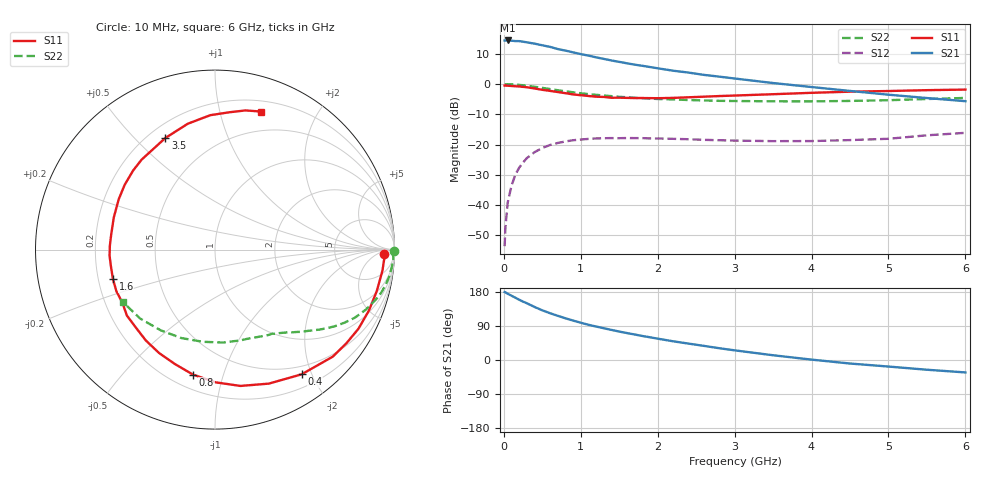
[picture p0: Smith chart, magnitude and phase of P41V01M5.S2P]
! SIEMENS Small Signal Semiconductors
! BFP182
! Si NPN RF Bipolar Junction Transistor in SOT143
! VCE = 1 V  IC = 1.5 mA
! Common Emitter S-Parameters:  March  1996
# GHz  S  MA  R  50
!  f  S11  S21  S12  S22
! GHz  MAG  ANG  MAG  ANG  MAG  ANG  MAG  ANG
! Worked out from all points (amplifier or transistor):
!   36 points, 10 MHz to 6 GHz, reference 50 ohm
!   highest |S21| = 14.4 dB at 50 MHz (marker M1)
!   |S21| within 3 dB of that: start of sweep to 732.6 MHz
!   unconditionally stable (mu >= 1): 2.318 GHz to end of sweep
!   at 250 MHz: K = 0.12, MSG = 20.0 dB, |S12| = -25.9 dB
!   at 1.4 GHz: K = 0.63, MSG = 12.8 dB, |S12| = -17.8 dB
!   at 6 GHz: K = 1.13, MAG = 3.1 dB, |S12| = -16.1 dB
!   S11 on the Smith chart (normalised r, x): 10 MHz: 29, -13; 400 MHz: 0.38, -1.85; 800 MHz: 0.29, -0.80; 1.6 GHz: 0.26, -0.13; 3.5 GHz: 0.27, +0.62; 6 GHz: 0.30, +1.35
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0.01  0.9437 -1.5  5.24 179.3  0.0021 89.0  0.9966 -0.6
0.02  0.9444 -3.0  5.253 178.6  0.0042 86.7  0.9914 -1.2
0.05  0.9403 -7.2  5.259 174.8  0.011 87.3  0.9954 -3.0
0.1  0.9305 -14.4  5.21 169.6  0.0211 80.9  0.9892 -5.9
0.2  0.9128 -28.9  5.129 159.0  0.0417 73.1  0.9709 -11.7
0.25  0.8989 -35.6  5.014 154.0  0.0507 68.4  0.9562 -14.6
0.4  0.8461 -55.2  4.653 139.9  0.0751 57.7  0.9037 -21.8
0.5  0.8047 -68.1  4.376 131.1  0.0881 50.7  0.8663 -26.0
0.6  0.7728 -79.4  4.123 123.5  0.0986 44.8  0.8278 -29.5
0.7  0.7397 -89.7  3.797 116.7  0.1064 39.7  0.7923 -32.6
0.8  0.7075 -99.9  3.575 110.1  0.1127 34.9  0.7605 -35.2
0.9  0.6756 -109.3  3.345 104.1  0.1182 31.1  0.7323 -37.5
1.1  0.6362 -127.3  2.954 92.9  0.1243 24.0  0.6835 -41.6
1.3  0.6132 -143.2  2.606 83.8  0.1276 18.3  0.6466 -45.2
1.6  0.5919 -163.8  2.206 71.1  0.1285 12.1  0.6063 -49.7
1.8  0.5884 -176.7  2.007 63.4  0.128 9.4  0.5861 -52.6
2.2  0.5916 162.4  1.664 49.4  0.1247 4.8  0.5581 -59.1
2.8  0.6342 136.0  1.328 31.1  0.1183 2.0  0.5287 -70.0
3.5  0.6805 114.0  1.041 12.5  0.1141 2.1  0.5196 -85.2
4.5  0.7494 92.0  0.771 -9.3  0.1188 6.9  0.5272 -110.8
5.5  0.7937 77.7  0.588 -25.7  0.1425 10.7  0.567 -137.4
6  0.8113 71.4  0.522 -32.8  0.1566 8.8  0.5903 -150.2
